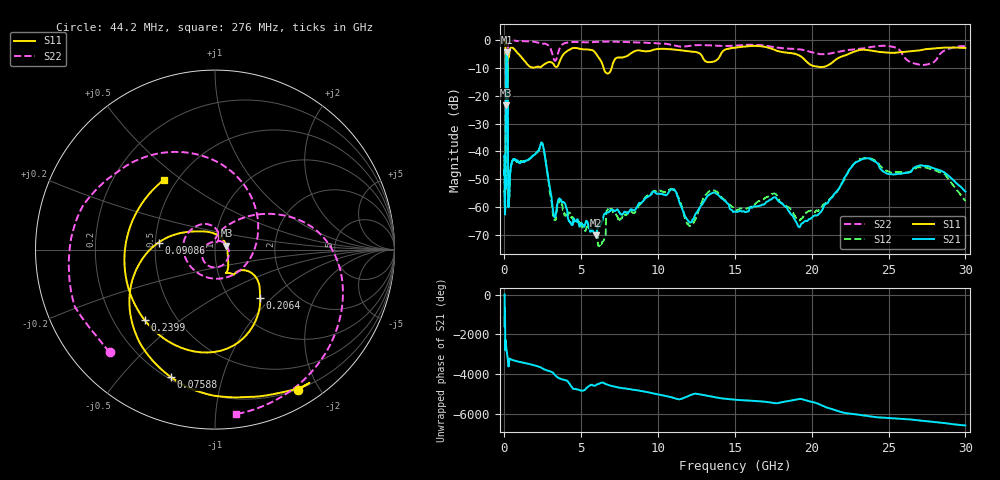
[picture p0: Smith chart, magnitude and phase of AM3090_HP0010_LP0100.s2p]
! Date/Time: Thu, Feb 28, 2019 1:55 PM
! Network Analyzer: Agilent Technologies E8364B Rev: A.07.50.67
! Sweep from 0.010 to 30.000 GHz, 1601 Points, Sweep Type: LOG
! Power Supply: 5.023 V, 0.002 A
# Hz S DB R 50
!freq MagS11 AngS11 MagS21 AngS21 MagS12 AngS12 MagS22 AngS22
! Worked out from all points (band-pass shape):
!   1601 points, 10 MHz to 30 GHz, reference 50 ohm
!   highest |S21| = -4.43 dB at 142.6 MHz (marker M1); lowest = -70.2 dB at 5.929 GHz (marker M2)
!   |S21| within 3 dB of the highest: 100.8 MHz to 196.4 MHz (95.61 MHz wide, 64.3 % of centre)
!   lowest |S11| = -23.4 dB at 99.43 MHz (marker M3), VSWR 1.14, Z = 56.8 + j2.4 ohm
!   |S11| at or under -10 dB: 90.88 MHz to 199.7 MHz (108.8 MHz wide, 74.9 % of centre); 6.451 GHz to 6.979 GHz (527.8 MHz wide, 7.86 % of centre)
!   |S22| runs from -28.3 to -0.2 dB; largest |S21 - S12| = 0.013
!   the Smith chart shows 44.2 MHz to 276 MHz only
!   S11 on the Smith chart (normalised r, x): 44.2 MHz: 0.19, -1.73; 75.88 MHz: 0.21, -0.69; 90.86 MHz: 0.52, +0.05; 206.4 MHz: 1.37, -0.85; 239.9 MHz: 0.33, -0.37; 276 MHz: 0.43, +0.43
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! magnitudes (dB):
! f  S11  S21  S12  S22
! 10 MHz  -0.3  -42.1  -47.1  -0.6
! 38.04 MHz  -0.5  -62.0  -59.4  -1.4
! 44.2 MHz  -0.8  -57.4  -59.0  -1.7
! 75.88 MHz  -2.5  -46.3  -48.0  -4.6
! 90.86 MHz  -10.0  -15.9  -15.9  -15.5
! 99.43 MHz  -23.4  -7.9  -7.9  -15.0
! 142.6 MHz  -15.8  -4.4  -4.4  -23.2
! 144.7 MHz  -15.7  -4.4  -4.4  -22.6
! 185.8 MHz  -13.9  -5.9  -5.9  -26.9
! 206.4 MHz  -8.7  -10.9  -10.9  -13.6
! 239.9 MHz  -5.1  -54.7  -53.8  -1.7
! 276 MHz  -6.3  -58.2  -57.2  -0.7
! 550.5 MHz  -2.9  -43.1  -43.0  -0.2
! 2.084 GHz  -9.7  -40.4  -40.6  -0.8
! 2.507 GHz  -9.1  -37.9  -37.9  -1.3
! 3.236 GHz  -9.0  -63.3  -63.9  -7.2
! 5.929 GHz  -4.6  -70.2  -66.0  -0.7
! 7.926 GHz  -5.9  -61.8  -62.9  -0.7
! 10.65 GHz  -3.3  -55.1  -54.3  -1.5
! 19.61 GHz  -7.5  -64.9  -62.2  -3.8
! 23.48 GHz  -3.5  -42.6  -42.4  -2.9
! 30 GHz  -2.9  -54.4  -57.8  -2.2
